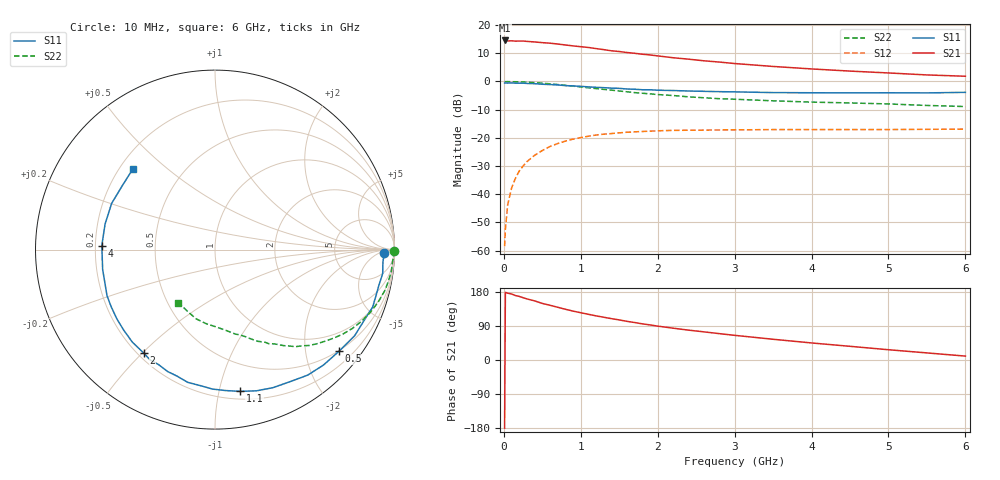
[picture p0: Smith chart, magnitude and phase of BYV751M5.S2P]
! SIEMENS Small Signal Semiconductors
! BFY420
! Si NPN RF SIEGET Grounded Emitter Transistor in MICRO-X
! VCE = 0.75 V  IC = 1.5 mA
! Common Emitter S-Parameters:  October  1996
# GHz  S  MA  R  50
!  f  S11  S21  S12  S22
! GHz  MAG  ANG  MAG  ANG  MAG  ANG  MAG  ANG
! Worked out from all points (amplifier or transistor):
!   36 points, 10 MHz to 6 GHz, reference 50 ohm
!   highest |S21| = 14.6 dB at 10 MHz (marker M1)
!   |S21| within 3 dB of that: start of sweep to 1.23 GHz
!   unconditionally stable (mu >= 1): 4.213 GHz to end of sweep
!   at 250 MHz: K = 0.05, MSG = 22.2 dB, |S12| = -30.0 dB
!   at 1.4 GHz: K = 0.28, MSG = 14.7 dB, |S12| = -18.5 dB
!   at 6 GHz: K = 1.30, MAG = 6.1 dB, |S12| = -16.9 dB
!   S11 on the Smith chart (normalised r, x): 10 MHz: 30, -9; 500 MHz: 0.48, -2.72; 1.1 GHz: 0.26, -1.16; 2 GHz: 0.22, -0.51; 4 GHz: 0.23, +0.02; 6 GHz: 0.25, +0.39
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0.01  0.9407 -1.1  5.343 -179.6  0.0012 106.5  0.9957 -0.4
0.02  0.9414 -2.0  5.319 178.5  0.0024 88.7  0.9922 -0.9
0.05  0.9382 -4.2  5.229 176.4  0.0065 86.9  0.9948 -2.3
0.1  0.9438 -8.1  5.269 174.2  0.0128 84.9  0.9904 -4.6
0.15  0.9348 -12.0  5.199 170.1  0.0191 81.8  0.9899 -7.0
0.2  0.933 -16.1  5.216 167.8  0.0258 81.0  0.9848 -9.1
0.25  0.9349 -20.0  5.215 164.4  0.0316 77.5  0.9788 -11.4
0.4  0.9141 -31.7  5.028 156.0  0.0491 70.5  0.9548 -17.9
0.5  0.8933 -39.4  4.888 149.3  0.0596 66.0  0.9326 -22.2
0.6  0.8825 -46.8  4.776 144.4  0.0704 61.6  0.9086 -26.1
0.8  0.8456 -60.7  4.44 133.9  0.0876 53.0  0.8543 -33.4
1.1  0.8023 -79.9  4.01 120.6  0.1071 42.7  0.7733 -42.7
1.4  0.7622 -96.2  3.499 109.1  0.1193 34.1  0.7027 -50.3
1.6  0.7359 -106.7  3.264 102.0  0.1259 29.5  0.6571 -54.5
2  0.7002 -124.5  2.846 89.4  0.1334 21.8  0.5867 -61.6
2.2  0.6912 -131.8  2.638 84.0  0.1358 18.3  0.5637 -65.0
2.8  0.6602 -151.1  2.211 69.6  0.1382 11.1  0.4951 -73.7
3.5  0.6356 -170.0  1.848 54.7  0.1404 5.4  0.4541 -82.3
4  0.6311 178.0  1.67 45.0  0.1403 2.2  0.4306 -89.2
4.5  0.6287 166.9  1.529 36.1  0.1405 -0.7  0.4166 -96.4
5.5  0.6276 145.0  1.307 18.7  0.1417 -3.9  0.3758 -114.2
6  0.6418 135.3  1.239 10.3  0.1431 -4.5  0.3593 -124.5
